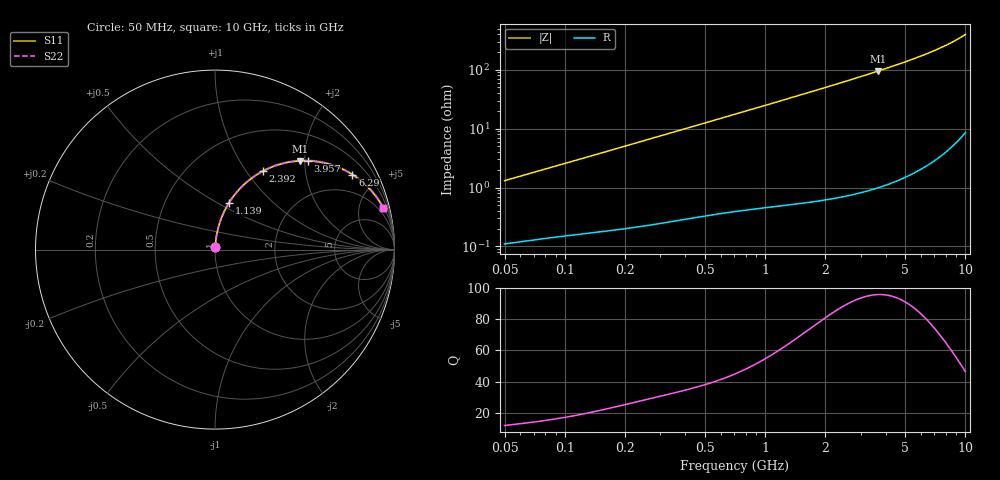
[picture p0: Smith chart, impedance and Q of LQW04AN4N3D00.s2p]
!Murata Part Number: LQW04AN4N3D00
!These Parameters are Measured in Series Mode Connection
!  o--[Z]--o
!Port1  Port2
!  o-------o
!Freq. Start=50[MHz] Stop=10[GHz], 401[Steps]
# Hz S RI R 50
!Freq.(Hz)	S 11(Real)	S 11(Imag)	S 21(Real)	S 21(Imag)	S 12(Real)	S 12(Imag)	S 22(Real)	S 22(Imag)
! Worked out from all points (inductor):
!   401 points, 50 MHz to 10 GHz, reference 50 ohm
!   read as one part in series: L = 4.13 nH near 51.34 MHz
!   highest Q = 95.8 at 3.654 GHz (marker M1), where L = 4.12 nH
!   S11 on the Smith chart (normalised r, x): 50 MHz: 1.00, +0.03; 1.139 GHz: 1.01, +0.57; 2.392 GHz: 1.01, +1.20; 3.957 GHz: 1.02, +2.07; 6.29 GHz: 1.04, +3.64; 10 GHz: 1.17, +7.93
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5e7  0.00127 0.013  0.9987 -0.013  0.9987 -0.013  0.00127 0.013
1.214486e8  0.00258 0.0308  0.9974 -0.0308  0.9974 -0.0308  0.00258 0.0308
1.956524e8  0.0044 0.0491  0.9956 -0.0491  0.9956 -0.0491  0.0044 0.0491
2.949953e8  0.00786 0.0733  0.9921 -0.0733  0.9921 -0.0733  0.00786 0.0733
4.689809e8  0.0166 0.1148  0.9834 -0.1148  0.9834 -0.1148  0.0166 0.1148
7.071068e8  0.0335 0.1692  0.9665 -0.1692  0.9665 -0.1692  0.0335 0.1692
9.094607e8  0.0522 0.213  0.9478 -0.213  0.9478 -0.213  0.0522 0.213
1.139142e9  0.0777 0.2594  0.9223 -0.2594  0.9223 -0.2594  0.0777 0.2594
1.408053e9  0.1126 0.3088  0.8874 -0.3088  0.8874 -0.3088  0.1126 0.3088
1.717543e9  0.158 0.3582  0.842 -0.3582  0.842 -0.3582  0.158 0.3582
2.040286e9  0.2095 0.4009  0.7905 -0.4009  0.7905 -0.4009  0.2095 0.4009
2.391784e9  0.2681 0.4373  0.7319 -0.4373  0.7319 -0.4373  0.2681 0.4373
2.99582e9  0.3691 0.4773  0.6309 -0.4773  0.6309 -0.4773  0.3691 0.4773
3.654301e9  0.4728 0.4941  0.5272 -0.4941  0.5272 -0.4941  0.4728 0.4941
3.956578e9  0.5166 0.4945  0.4834 -0.4945  0.4834 -0.4945  0.5166 0.4945
4.171863e9  0.5462 0.4926  0.4538 -0.4926  0.4538 -0.4926  0.5462 0.4926
5.088839e9  0.6564 0.4694  0.3436 -0.4694  0.3436 -0.4694  0.6564 0.4694
6.290134e9  0.7653 0.4177  0.2347 -0.4177  0.2347 -0.4177  0.7653 0.4177
7.086521e9  0.8192 0.3781  0.1808 -0.3781  0.1808 -0.3781  0.8192 0.3781
7.983737e9  0.8665 0.3325  0.1335 -0.3325  0.1335 -0.3325  0.8665 0.3325
8.759398e9  0.8983 0.2937  0.1017 -0.2937  0.1017 -0.2937  0.8983 0.2937
1e10  0.9358 0.2345  0.0642 -0.2345  0.0642 -0.2345  0.9358 0.2345
